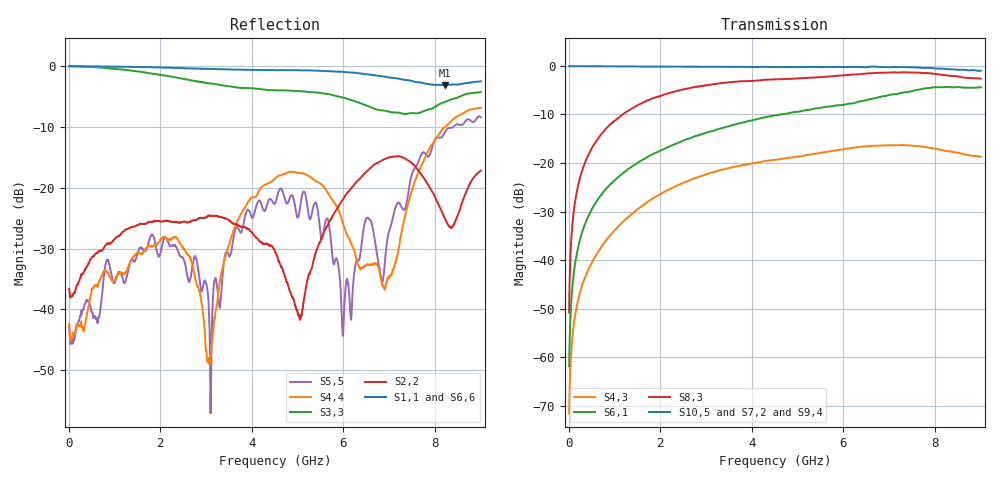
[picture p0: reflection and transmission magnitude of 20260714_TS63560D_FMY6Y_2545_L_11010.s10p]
# GHz S DB R 50
! CMT, SN0916, 25263762, 26.7.0
! Date: 15.07.2026 13:47:56
! Data: Format
! Freq S1.1:dB/Ang S1.2:dB/Ang S1.3:dB/Ang S1.4:dB/Ang S1.5:dB/Ang S1.6:dB/Ang S1.7:dB/Ang S1.8:dB/Ang S1.9:dB/Ang S1.10:dB/Ang
!  S2.1:dB/Ang S2.2:dB/Ang S2.3:dB/Ang S2.4:dB/Ang S2.5:dB/Ang S2.6:dB/Ang S2.7:dB/Ang S2.8:dB/Ang S2.9:dB/Ang S2.10:dB/Ang
!  S3.1:dB/Ang S3.2:dB/Ang S3.3:dB/Ang S3.4:dB/Ang S3.5:dB/Ang S3.6:dB/Ang S3.7:dB/Ang S3.8:dB/Ang S3.9:dB/Ang S3.10:dB/Ang
!  S4.1:dB/Ang S4.2:dB/Ang S4.3:dB/Ang S4.4:dB/Ang S4.5:dB/Ang S4.6:dB/Ang S4.7:dB/Ang S4.8:dB/Ang S4.9:dB/Ang S4.10:dB/Ang
!  S5.1:dB/Ang S5.2:dB/Ang S5.3:dB/Ang S5.4:dB/Ang S5.5:dB/Ang S5.6:dB/Ang S5.7:dB/Ang S5.8:dB/Ang S5.9:dB/Ang S5.10:dB/Ang
!  S6.1:dB/Ang S6.2:dB/Ang S6.3:dB/Ang S6.4:dB/Ang S6.5:dB/Ang S6.6:dB/Ang S6.7:dB/Ang S6.8:dB/Ang S6.9:dB/Ang S6.10:dB/Ang
!  S7.1:dB/Ang S7.2:dB/Ang S7.3:dB/Ang S7.4:dB/Ang S7.5:dB/Ang S7.6:dB/Ang S7.7:dB/Ang S7.8:dB/Ang S7.9:dB/Ang S7.10:dB/Ang
!  S8.1:dB/Ang S8.2:dB/Ang S8.3:dB/Ang S8.4:dB/Ang S8.5:dB/Ang S8.6:dB/Ang S8.7:dB/Ang S8.8:dB/Ang S8.9:dB/Ang S8.10:dB/Ang
!  S9.1:dB/Ang S9.2:dB/Ang S9.3:dB/Ang S9.4:dB/Ang S9.5:dB/Ang S9.6:dB/Ang S9.7:dB/Ang S9.8:dB/Ang S9.9:dB/Ang S9.10:dB/Ang
!  S10.1:dB/Ang S10.2:dB/Ang S10.3:dB/Ang S10.4:dB/Ang S10.5:dB/Ang S10.6:dB/Ang S10.7:dB/Ang S10.8:dB/Ang S10.9:dB/Ang S10.10:dB/Ang
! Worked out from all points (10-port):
!   2001 points, 10 MHz to 9 GHz, reference 50 ohm
!   strongest paths, dB at 10 MHz, 2.257 GHz, 4.505 GHz, 6.753 GHz, 9 GHz:
!     S10,5: -0.1, -0.2, -0.2, -0.2, -1.0
!     S7,2: -0.1, -0.2, -0.3, -0.6, -0.6
!     S9,4: -0.1, -0.2, -0.4, -0.4, -1.5
!     S8,3: -50.8, -5.5, -2.8, -1.4, -2.6
!     S6,1: -61.9, -16.4, -10.2, -6.5, -4.4
!     S4,3: -71.6, -25.2, -19.4, -16.4, -18.7
!   lowest |S11| = -3.1 dB at 8.213 GHz (marker M1), VSWR 5.62, Z = 11 - j23.8 ohm
!   |S11| at or under -10 dB: nowhere
